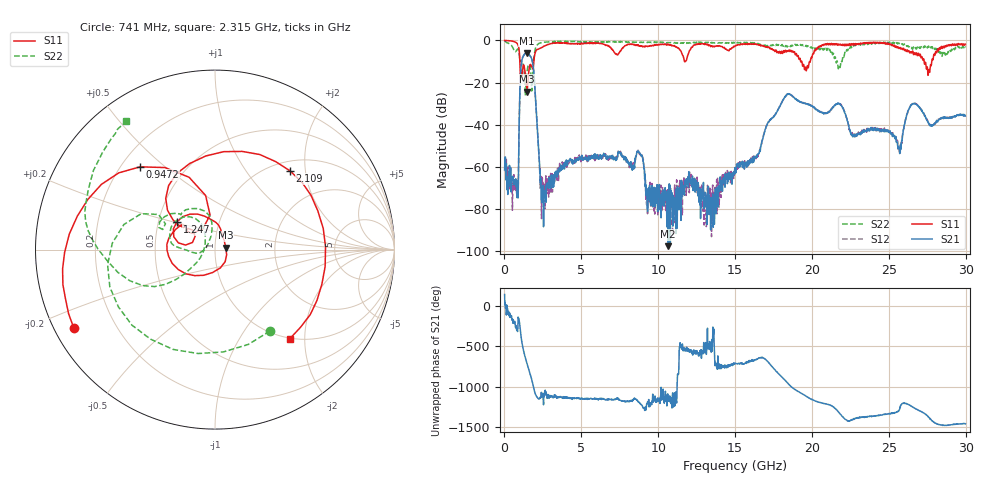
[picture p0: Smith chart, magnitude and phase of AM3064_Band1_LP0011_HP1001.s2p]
# Hz S DB R 50.0
!freq dBS11 angS11 dBS21 angS21 dBS12 angS12 dBS22 angS22
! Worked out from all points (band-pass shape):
!   1600 points, 10 MHz to 29.98 GHz, reference 50 ohm
!   highest |S21| = -5.97 dB at 1.435 GHz (marker M1); lowest = -97.6 dB at 10.66 GHz (marker M2)
!   |S21| within 3 dB of the highest: 1.149 GHz to 1.781 GHz (631.2 MHz wide, 43.1 % of centre)
!   lowest |S11| = -24.2 dB at 1.472 GHz (marker M3), VSWR 1.13, Z = 56.4 + j1.24 ohm
!   |S11| at or under -10 dB: 1.002 GHz to 1.913 GHz (911.6 MHz wide, 62.6 % of centre); 19.34 GHz to 19.89 GHz (546.2 MHz wide, 2.78 % of centre); 27.3 GHz to 27.79 GHz (495.2 MHz wide, 1.8 % of centre)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
!   |S22| runs from -26.1 to -0.3 dB; largest |S21 - S12| = 0.0066
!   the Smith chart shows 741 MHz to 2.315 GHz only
!   S11 on the Smith chart (normalised r, x): 741 MHz: 0.06, -0.26; 947.2 MHz: 0.28, +0.41; 1.247 GHz: 0.62, +0.21; 2.109 GHz: 1.19, +1.65; 2.315 GHz: 0.98, -1.69
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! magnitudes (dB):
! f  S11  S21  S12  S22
! 10 MHz  0.0  -61.4  -56.4  -0.3
! 741 MHz  -0.9  -65.7  -71.2  -5.2
! 947.2 MHz  -4.1  -43.7  -43.8  -5.6
! 1.247 GHz  -11.6  -7.2  -7.1  -12.1
! 1.435 GHz  -20.6  -6.0  -5.9  -17.6
! 1.472 GHz  -24.2  -6.0  -6.0  -14.9
! 1.828 GHz  -13.4  -10.4  -10.3  -17.7
! 2.109 GHz  -4.4  -38.4  -38.2  -2.3
! 2.315 GHz  -3.8  -61.5  -60.9  -1.2
! 2.559 GHz  -2.7  -75.4  -70.7  -0.8
! 5.015 GHz  -1.5  -55.7  -56.3  -0.8
! 8.763 GHz  -2.7  -53.0  -53.8  -1.0
! 9.307 GHz  -2.8  -81.1  -82.2  -1.0
! 10 GHz  -2.0  -72.2  -72.4  -0.9
! 10.66 GHz  -2.1  -97.6  -82.9  -1.0
! 13.52 GHz  -3.0  -79.0  -73.0  -1.2
! 15 GHz  -2.7  -63.0  -62.1  -1.3
! 18.36 GHz  -5.3  -25.7  -25.7  -2.9
! 19.99 GHz  -8.3  -31.2  -31.2  -3.4
! 25 GHz  -1.5  -43.3  -43.2  -1.0
! 27.56 GHz  -16.4  -39.2  -38.7  -2.9
! 29.98 GHz  -1.8  -35.9  -35.2  -3.3
